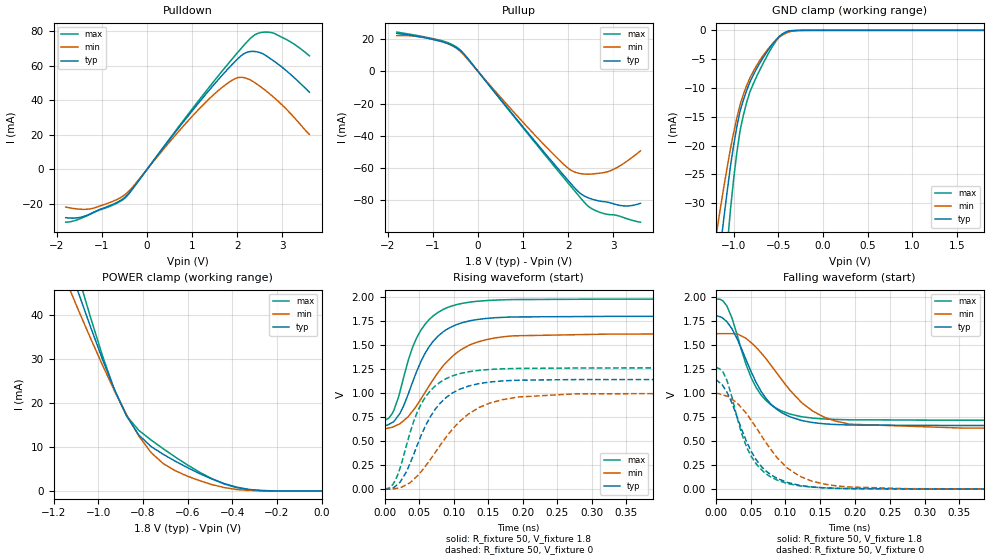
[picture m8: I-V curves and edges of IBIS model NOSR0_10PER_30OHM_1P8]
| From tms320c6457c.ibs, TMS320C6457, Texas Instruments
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|   Model Cell NOSR0_10PER_30OHM_1P8
|NOSR0_10PER_30OHM_1P8
[Model]   NOSR0_10PER_30OHM_1P8
Model_type   3-state
Polarity   Non-Inverting
Enable   Active-Low
Cref =  15.0000pF
Rref =  100.0000M
Vref =  0V
Vmeas =  0.9
C_comp   1.89p   1.72p   2.18p
[Model Spec]
Rref 50 NA NA
Vref 0.9 0.81 0.99
[Temperature Range]   25   125   -40
[Voltage Range]   1.8   1.62   1.98
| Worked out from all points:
|   slope of the pulldown table from 0 to 0.27 V, typ, clamps not added: 28.9 ohm
|   slope of the pullup table from 0 to 0.27 V, typ, clamps not added: 28.7 ohm
|   GND clamp passes 1 mA (typ) near -0.48 V on its own axis
|   POWER clamp passes 1 mA (typ) near -0.39 V on its own axis
|   rising waveform, R_fixture 50, V_fixture 1.8: 20-80 % time 45.8ps typ, 62.7ps min, 39.3ps max; typ from 0.663 V to 1.8 V
|   rising waveform, R_fixture 50, V_fixture 0: 20-80 % time 48.7ps typ, 70.1ps min, 40.9ps max; typ from 0 V to 1.14 V
|   falling waveform, R_fixture 50, V_fixture 1.8: 20-80 % time 48.4ps typ, 71.7ps min, 40.8ps max; typ from 1.8 V to 0.663 V
|   falling waveform, R_fixture 50, V_fixture 0: 20-80 % time 44.4ps typ, 64.2ps min, 38.2ps max; typ from 1.14 V to 0.001 V
| Nom Voltages:
|   BIAS2=0.9, BIASFET=0, VDD=1.1, VDDS=1.8, BUS_BIAS1=0, BUS_BIAS3=0,
|   VSS=0, VSSS=0
| Min Voltages:
|   BIAS2=0.81, BIASFET=0, VDD=0.99, VDDS=1.62, BUS_BIAS1=0, BUS_BIAS3=0,
|   VSS=0, VSSS=0
| Max Voltages:
|   BIAS2=0.99, BIASFET=0, VDD=1.21, VDDS=1.98, BUS_BIAS1=0, BUS_BIAS3=0,
|   VSS=0, VSSS=0
[POWER_clamp]
|   voltage   I(typ)   I(min)   I(max)
-1.8V     156mA      133.5mA    181.7mA
-1.127V   50.87mA    45.88mA    55.74mA
-1.109V   48.19mA    43.68mA    52.51mA
-1.073V   42.88mA    39.33mA    46.15mA
-1.055V   40.27mA    37.18mA    43.01mA
-927.3mV  23.11mA    22.83mA    22.99mA
-872.7mV  17.08mA    17.31mA    17.08mA
-818.2mV  12.73mA    12.5mA     13.8mA
-763.6mV  10.13mA    8.758mA    11.61mA
-600mV    5.297mA    3.359mA    5.911mA
-381.8mV  881.1uA    334.9uA    769uA
0V        130.3nA    147.3nA    381.2nA
[Pulldown]
|   voltage   I(typ)   I(min)   I(max)
-1.8V     -27.85mA   -21.72mA   -30.44mA
-1.473V   -27.61mA   -22.95mA   -28.35mA
-1.2V     -24.94mA   -22.44mA   -25.12mA
-436.4mV  -14.77mA   -13.46mA   -15.19mA
1.145V    38.45mA    34.66mA    39.73mA
1.636V    53.5mA     46.78mA    55.86mA
2.018V    64.04mA    53.05mA    67.79mA
2.291V    68.15mA    51.72mA    75.67mA
2.455V    67.85mA    49mA       78.57mA
2.673V    65.14mA    44.71mA    79.32mA
3.164V    55.37mA    32.84mA    74mA
3.6V      44.58mA    20.25mA    65.64mA
[Pullup]
|   voltage   I(typ)   I(min)   I(max)
-1.8V     23.6mA     22.14mA    24.38mA
-927.3mV  19.33mA    19.47mA    19.84mA
-600mV    16.43mA    16.37mA    17mA
-381.8mV  12.59mA    12.15mA    12.97mA
1.309V    -44.94mA   -40.98mA   -45.82mA
1.909V    -64.81mA   -57.95mA   -66.32mA
2.127V    -71.85mA   -62.27mA   -73.67mA
2.291V    -76.19mA   -63.49mA   -79.14mA
2.455V    -78.54mA   -63.78mA   -83.94mA
2.891V    -81.27mA   -62.08mA   -88.79mA
3.273V    -83.51mA   -56.25mA   -91.14mA
3.6V      -81.85mA   -49.3mA    -93.55mA
[GND_clamp]
|   voltage   I(typ)   I(min)   I(max)
-1.8V     -137.1mA   -107.1mA   -189.7mA
-1.182V   -42.18mA   -34.28mA   -58.62mA
-1.109V   -32.61mA   -27.18mA   -44.51mA
-1.073V   -28.08mA   -23.86mA   -37.8mA
-1.036V   -23.72mA   -20.65mA   -31.33mA
-963.6mV  -16.74mA   -15.21mA   -21.21mA
-927.3mV  -13.99mA   -12.88mA   -17.38mA
-854.5mV  -10.47mA   -9.599mA   -12.54mA
-781.8mV  -7.837mA   -7.198mA   -9.373mA
-600mV    -3.116mA   -2.961mA   -3.703mA
-418.2mV  -354.7uA   -522.3uA   -297.6uA
1.8V      130.3nA    2.912uA    201.9nA
[Ramp]
| variable   typ   min   max
dV/dt_f 0.57400245/38.505318p 0.50413553/57.182635p  0.6346154/31.922539p
dV/dt_r 0.57484742/38.272521p  0.5033393/55.78909p  0.63492598/31.990085p
R_load = 50
[Rising Waveform]
R_fixture = 50
V_fixture = 1.8
V_fixture_min = 1.62
V_fixture_max = 1.98
|   time   V(typ)   V(min)   V(max)
0s        663.1mV    628.6mV    717mV
11.4ps    695.8mV    645mV      791.7mV
22.14ps   788.7mV    681.4mV    1.013V
40.14ps   1.108V     810.1mV    1.471V
58.14ps   1.409V     1.002V     1.713V
84.94ps   1.639V     1.286V     1.872V
123.9ps   1.754V     1.504V     1.948V
186.4ps   1.793V     1.597V     1.974V
323.6ps   1.799V     1.615V     1.979V
1.181ns   1.8V       1.62V      1.98V
[Rising Waveform]
R_fixture = 50
V_fixture = 0
V_fixture_min = 0
V_fixture_max = 0
|   time   V(typ)   V(min)   V(max)
0s        0V         586.1uV    973.9uV
11.9ps    13.81mV    649.1uV    47.26mV
22.14ps   70.12mV    13.95mV    212.6mV
42.04ps   361.4mV    102mV      705mV
58.74ps   653.3mV    236.2mV    955.3mV
88.54ps   951.3mV    537.9mV    1.15V
121.7ps   1.074V     784.4mV    1.223V
170.8ps   1.127V     932.5mV    1.253V
277.9ps   1.141V     993mV      1.262V
1.179ns   1.142V     998mV      1.264V
[Falling Waveform]
R_fixture = 50
V_fixture = 1.8
V_fixture_min = 1.62
V_fixture_max = 1.98
|   time   V(typ)   V(min)   V(max)
0s        1.799V     1.62V      1.98V
15.94ps   1.746V     1.62V      1.908V
23.44ps   1.667V     1.62V      1.779V
44.14ps   1.338V     1.567V     1.287V
65.14ps   1.019V     1.42V      980.7mV
86.24ps   839.8mV    1.224V     845.8mV
123ps     715.9mV    903.9mV    755.1mV
155.2ps   681.3mV    751.8mV    731.7mV
192.4ps   668.5mV    677.1mV    722.7mV
1.181ns   663.2mV    629.6mV    717.9mV
[Falling Waveform]
R_fixture = 50
V_fixture = 0
V_fixture_min = 0
V_fixture_max = 0
|   time   V(typ)   V(min)   V(max)
0s        1.143V     999.6mV    1.264V
10.5ps    1.074V     981.8mV    1.22V
15.64ps   1.017V     970.3mV    1.141V
37.04ps   625.9mV    846.8mV    583.2mV
58.14ps   306.1mV    641.3mV    264.2mV
88.84ps   110.1mV    321.9mV    92.59mV
120.3ps   40.46mV    136mV      35.22mV
174ps     8.677mV    34.05mV    10.11mV
278.2ps   2.397mV    5.556mV    3.653mV
1.179ns   944.4uV    1.019mV    604.2uV
